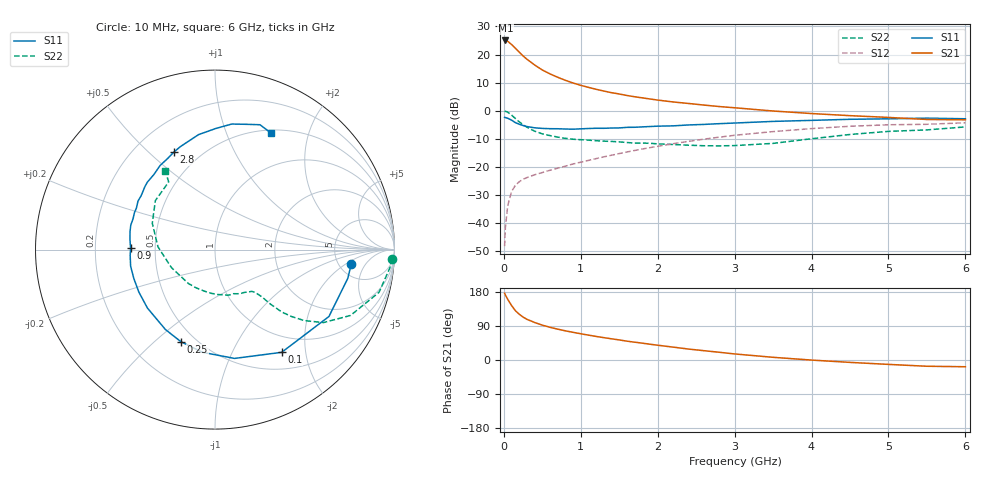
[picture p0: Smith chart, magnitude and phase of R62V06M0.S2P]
! SIEMENS Small Signal Semiconductors
! BFR193
! Si NPN RF Bipolar Junction Transistor in SOT23
! VCE = 2 V  IC = 6 mA
! Common Emitter S-Parameters:  May  1996
# GHz  S  MA  R  50
!  f  S11  S21  S12  S22
! GHz  MAG  ANG  MAG  ANG  MAG  ANG  MAG  ANG
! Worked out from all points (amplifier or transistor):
!   36 points, 10 MHz to 6 GHz, reference 50 ohm
!   highest |S21| = 25.0 dB at 20 MHz (marker M1)
!   |S21| within 3 dB of that: start of sweep to 158.9 MHz
!   unconditionally stable (mu >= 1): 826.3 MHz to 1.976 GHz
!   at 250 MHz: K = 0.49, MSG = 22.0 dB, |S12| = -24.4 dB
!   at 1.4 GHz: K = 1.06, MAG = 9.6 dB, |S12| = -15.8 dB
!   at 6 GHz: K = 0.97, MSG = 0.5 dB, |S12| = -4.3 dB
!   lowest NFmin = 1.20 dB at 450 MHz
!   S11 on the Smith chart (normalised r, x): 10 MHz: 6.42, -2.54; 100 MHz: 0.74, -1.58; 250 MHz: 0.42, -0.61; 900 MHz: 0.36, +0.01; 2.8 GHz: 0.36, +0.60; 6 GHz: 0.53, +1.45
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0.01  0.7632 -6.2  17.7 176.2  0.0039 87.6  0.9882 -2.9
0.02  0.7571 -12.2  17.84 171.7  0.0084 83.6  0.9795 -6.0
0.05  0.7362 -30.4  17.25 160.3  0.0203 74.8  0.9445 -14.6
0.1  0.6824 -57.0  15.13 143.9  0.0365 64.6  0.8396 -25.9
0.15  0.616 -79.8  13 130.1  0.0472 56.7  0.7288 -33.9
0.2  0.5764 -97.0  11.06 120.8  0.0546 52.4  0.6355 -38.5
0.25  0.5472 -110.3  9.456 113.3  0.0603 49.8  0.5657 -41.2
0.3  0.524 -121.8  8.275 107.4  0.0648 49.1  0.5108 -43.0
0.4  0.4978 -139.1  6.539 99.0  0.0726 49.3  0.4341 -44.5
0.5  0.4858 -150.9  5.316 92.0  0.0797 50.1  0.3888 -45.0
0.6  0.48 -160.5  4.53 86.3  0.0874 51.3  0.3618 -45.5
0.7  0.4791 -168.9  3.948 81.4  0.0951 53.2  0.3405 -46.3
0.9  0.4703 179.0  3.124 73.0  0.113 56.0  0.3117 -48.4
1.1  0.484 168.0  2.611 65.7  0.131 57.5  0.3002 -52.1
1.3  0.488 159.2  2.244 59.0  0.1515 58.4  0.2882 -56.1
1.6  0.5073 147.7  1.871 49.7  0.1849 58.5  0.2727 -64.4
2.2  0.5392 129.2  1.436 34.0  0.2595 55.1  0.2513 -85.8
2.8  0.59 112.8  1.19 20.4  0.3393 48.3  0.2377 -116.2
3.5  0.6473 98.1  0.991 7.1  0.4264 37.4  0.2631 -157.9
4.5  0.7058 82.4  0.819 -6.3  0.5302 21.4  0.379 157.2
5.5  0.7394 70.2  0.7 -16.5  0.575 4.9  0.4569 124.4
6  0.721 64.5  0.691 -17.8  0.6121 0.1  0.5168 122.3
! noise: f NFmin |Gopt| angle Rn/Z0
0.45  1.2  0.25  114  0.13
0.9  1.25  0.37  150  0.12
1.8  2  0.55  -158  0.12
